TYPE E_IEC870_5_101SState :
(
	e101SState_Init := 0,

	e101SState_TestAct,
	e101SState_TestCon,

	e101SState_ClockAct,
	e101SState_ClockSet,
	e101SState_ClockCon,

	e101SState_GeninAct,
	e101SState_GeninCon,
	e101SState_GeninTerm,

	e101SState_CoroAct,
	e101SState_CoroCon,
	e101SState_CoroTerm,

	e101SState_DelayAct,
	e101SState_DelayCon,
	e101SState_DelaySpt,
	
	e101SState_ScsCmdAct,
	e101SState_DcsCmdAct,
	e101SState_RcsCmdAct,
	e101SState_BsiCmdAct,
	e101SState_NvaCmdAct,
	e101SState_SvaCmdAct,
	e101SState_R32CmdAct,
	
	e101SState_GenCmdSel,
	e101SState_GenCmdCon,
	e101SState_GenCmdExe,
	e101SState_GenCmdTerm
);
END_TYPE
